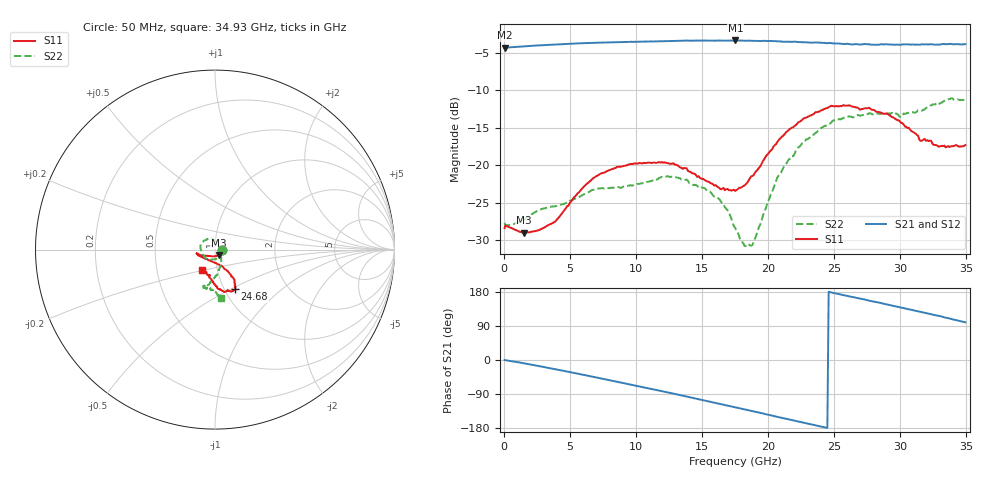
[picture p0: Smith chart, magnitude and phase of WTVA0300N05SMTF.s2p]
! 50 ohm 2-Port S-parameters measured by Modelithics Inc support@modelithics.com  Tampa, FL USA 813-866-6335 (February 2024)
! Smiths Interconnect,  3dB P/N: WTVA0300N05SMTF, Temperature: -25 C
! Board: 10 mil Rogers 4350B, Mounting Pad Dimensions: Length: 15 mils, Width: 25 mils, Gap: 40 mils.
# Hz S RI R 50
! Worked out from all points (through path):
!   352 points, 50 MHz to 34.93 GHz, reference 50 ohm
!   highest |S21| = -3.32 dB at 17.51 GHz (marker M1); lowest = -4.3 dB at 50 MHz (marker M2)
!   group delay of S21, straight-line fit = 21 ps
!   lowest |S11| = -29.0 dB at 1.494 GHz (marker M3), VSWR 1.07, Z = 51.9 - j3.08 ohm
!   |S11| at or under -10 dB: start of sweep to end of sweep
!   |S22| runs from -30.8 to -11.1 dB; largest |S21 - S12| = 0.0061
!   S11 on the Smith chart (normalised r, x): 50 MHz: 1.08, -0.00; 24.68 GHz: 1.12, -0.53; 34.93 GHz: 0.84, -0.20
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5e7  0.038 -0.00117  0.6109 -0.00196  0.6105 -0.00209  0.0412 -0.00118
1.4935e9  0.0195 -0.0297  0.6169 -0.0927  0.6165 -0.0927  0.0235 -0.0363
3.8815e9  -0.0216 -0.0361  0.5847 -0.2636  0.584 -0.264  -0.00148 -0.0532
5.8715e9  -0.0604 -0.0337  0.5138 -0.4035  0.5132 -0.4036  -0.0287 -0.0557
8.558e9  -0.0938 -0.0269  0.3591 -0.5587  0.358 -0.5588  -0.0605 -0.0384
1.1742e10  -0.1025 -0.0227  0.1096 -0.6645  0.1081 -0.6643  -0.0816 0.0112
1.38315e10  -0.0892 -0.0339  -0.0741 -0.6775  -0.075 -0.6771  -0.0634 0.0494
1.56225e10  -0.059 -0.0479  -0.2341 -0.6394  -0.2354 -0.6384  -0.0236 0.062
1.66175e10  -0.0411 -0.0574  -0.3175 -0.6019  -0.3188 -0.601  -0.00475 0.055
1.7513e10  -0.0181 -0.065  -0.3895 -0.56  -0.3906 -0.5588  0.012 0.0361
1.82095e10  -0.000304 -0.0734  -0.4394 -0.5179  -0.4403 -0.5167  0.0211 0.0198
1.88065e10  0.0185 -0.0829  -0.4808 -0.4791  -0.4813 -0.478  0.0293 -0.00188
2.0697e10  0.0736 -0.1234  -0.5839 -0.3362  -0.5846 -0.3342  0.0339 -0.0759
2.2289e10  0.1049 -0.1631  -0.634 -0.2016  -0.6344 -0.1995  0.016 -0.1309
2.33835e10  0.1097 -0.1889  -0.6517 -0.1076  -0.6516 -0.1063  -0.00604 -0.1591
2.4677e10  0.112 -0.2201  -0.6556 0.0104  -0.6554 0.0115  -0.0286 -0.1871
2.7662e10  0.0512 -0.2362  -0.5893 0.2581  -0.588 0.2602  -0.0652 -0.2133
2.91545e10  0.0156 -0.2165  -0.5261 0.3664  -0.5244 0.3681  -0.0507 -0.2166
3.005e10  -0.0037 -0.192  -0.4803 0.4195  -0.4787 0.421  -0.0304 -0.2068
3.15425e10  -0.0291 -0.1425  -0.3887 0.5094  -0.3874 0.5101  -0.00835 -0.2319
3.3831e10  -0.0615 -0.1188  -0.2049 0.6135  -0.2004 0.6147  0.037 -0.2774
3.49255e10  -0.0742 -0.1145  -0.1071 0.6354  -0.1023 0.6358  0.0347 -0.2701
